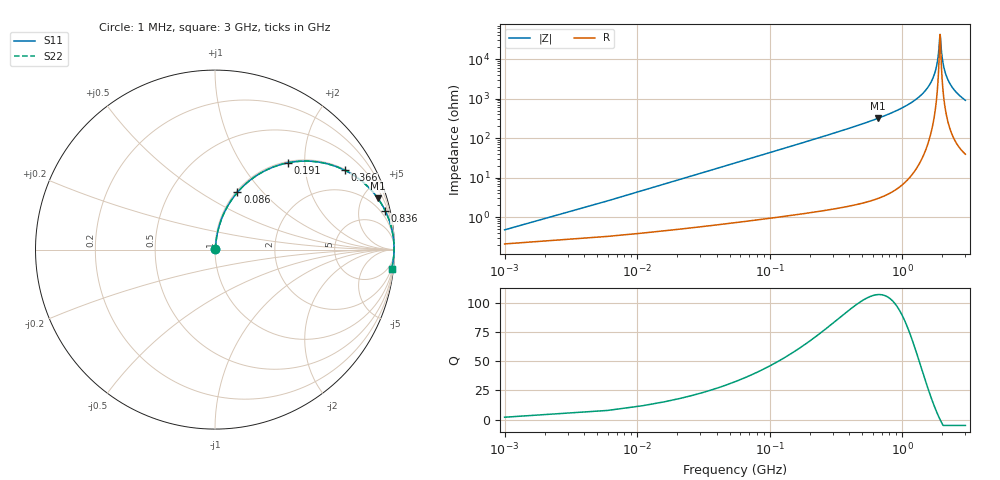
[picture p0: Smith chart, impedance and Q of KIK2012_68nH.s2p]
!version-2
!date-01.2022
!Series
# MHz S RI R 50
!Freq ReS11 ImS11 ReS21 ImS21 ReS12 ImS12 ReS22 ImS22
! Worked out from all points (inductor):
!   601 points, 1 MHz to 3 GHz, reference 50 ohm
!   read as one part in series: L = 68 nH near 16 MHz
!   highest Q = 107 at 656 MHz (marker M1), where L = 76.9 nH
!   self-resonance near 1.931 GHz
!   S11 on the Smith chart (normalised r, x): 1 MHz: 1.00, +0.01; 86 MHz: 1.02, +0.74; 191 MHz: 1.03, +1.65; 366 MHz: 1.04, +3.24; 836 MHz: 1.09, +8.79; 3 GHz: 2, -18
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1  0.00211 0.00425  0.9979 -0.00425  0.9979 -0.00425  0.00211 0.00425
21  0.0128 0.0881  0.9872 -0.0881  0.9872 -0.0881  0.0128 0.0881
31  0.0227 0.1287  0.9773 -0.1287  0.9773 -0.1287  0.0227 0.1287
51  0.0514 0.2054  0.9486 -0.2054  0.9486 -0.2054  0.0514 0.2054
86  0.1252 0.3193  0.8748 -0.3193  0.8748 -0.3193  0.1252 0.3193
191  0.4059 0.4835  0.5941 -0.4835  0.5941 -0.4835  0.4059 0.4835
366  0.7224 0.4423  0.2776 -0.4423  0.2776 -0.4423  0.7224 0.4423
501  0.838 0.3636  0.162 -0.3636  0.162 -0.3636  0.838 0.3636
656  0.9072 0.2855  0.0928 -0.2855  0.0928 -0.2855  0.9072 0.2855
836  0.9489 0.2154  0.0511 -0.2154  0.0511 -0.2154  0.9489 0.2154
1001  0.9698 0.1656  0.0302 -0.1656  0.0302 -0.1656  0.9698 0.1656
1501  0.9943 0.0614  0.00566 -0.0614  0.00566 -0.0614  0.9943 0.0614
1671  0.9967 0.0352  0.00326 -0.0352  0.00326 -0.0352  0.9967 0.0352
1791  0.9975 0.0184  0.0025 -0.0184  0.0025 -0.0184  0.9975 0.0184
1861  0.9977 0.0091  0.00234 -0.0091  0.00234 -0.0091  0.9977 0.0091
1931  0.9976 0.000203  0.00236 -0.000203  0.00236 -0.000203  0.9976 0.000203
1946  0.9976 -0.00166  0.00238 0.00166  0.00238 0.00166  0.9976 -0.00166
2001  0.9975 -0.00838  0.00254 0.00838  0.00254 0.00838  0.9975 -0.00838
2071  0.9971 -0.0167  0.00286 0.0167  0.00286 0.0167  0.9971 -0.0167
2171  0.9964 -0.028  0.00355 0.028  0.00355 0.028  0.9964 -0.028
2501  0.9926 -0.0624  0.00737 0.0624  0.00737 0.0624  0.9926 -0.0624
3000  0.9835 -0.1076  0.0165 0.1076  0.0165 0.1076  0.9835 -0.1076
